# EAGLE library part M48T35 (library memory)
5V, 256 Kbit (32 Kb x8) TIMEKEEPER® SRAM Source: http://www.st.com/stonline/books/pdf/docs/2611.pdf#search=%22M48T35%22
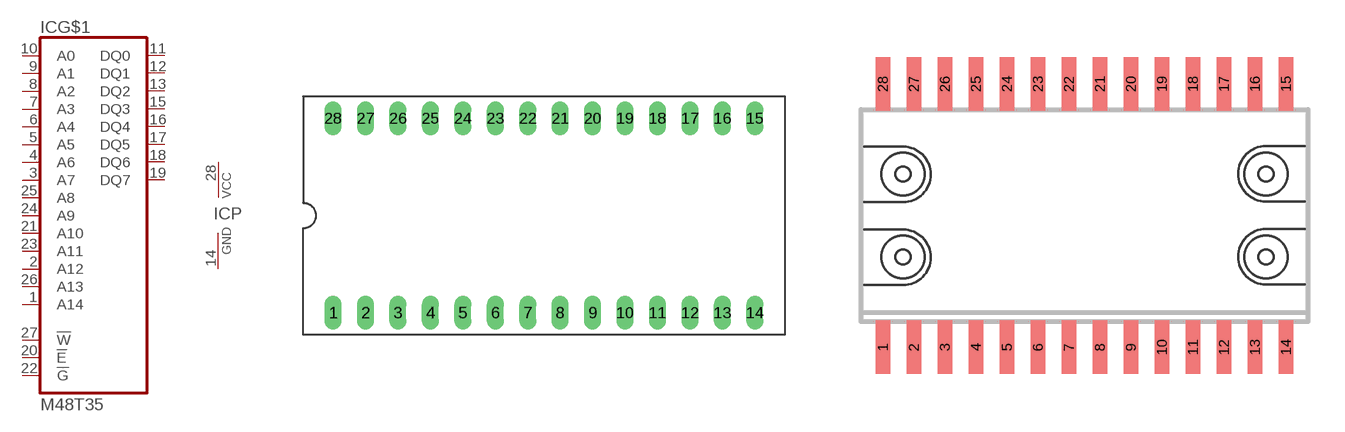
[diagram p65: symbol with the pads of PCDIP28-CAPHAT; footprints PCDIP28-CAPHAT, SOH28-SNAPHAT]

Designator prefix IC; gates G$1=M48T35 P=PWRN

## M48T35PC  [PCDIP28-CAPHAT]
1  G$1:A14  in
2  G$1:A12  in
3  G$1:A7  in
4  G$1:A6  in
5  G$1:A5  in
6  G$1:A4  in
7  G$1:A3  in
8  G$1:A2  in
9  G$1:A1  in
10  G$1:A0  in
11  G$1:DQ0
12  G$1:DQ1
13  G$1:DQ2
14  P:GND  pwr
15  G$1:DQ3
16  G$1:DQ4
17  G$1:DQ5
18  G$1:DQ6
19  G$1:DQ7
20  G$1:!E  in
21  G$1:A10  in
22  G$1:!G  in
23  G$1:A11  in
24  G$1:A9  in
25  G$1:A8  in
26  G$1:A13  in
27  G$1:!W  in
28  P:VCC  pwr

## M48T35MH  [SOH28-SNAPHAT]
Pads as for PCDIP28-CAPHAT

## Footprint PCDIP28-CAPHAT (pad centres in mm)
28-pin PCDIP, CAPHAT(TM) Package PCDIP28 (PC) Source: http://www.st.com/stonline/books/pdf/docs/2611.pdf#search=%22M48T35%22
drill 0.813 long: 1 -16.51,-7.62; 2 -13.97,-7.62; 3 -11.43,-7.62; 4 -8.89,-7.62; 5 -6.35,-7.62; 6 -3.81,-7.62; 7 -1.27,-7.62; 8 1.27,-7.62; 9 3.81,-7.62; 10 6.35,-7.62; 11 8.89,-7.62; 12 11.43,-7.62; 13 13.97,-7.62; 14 16.51,-7.62; 15 16.51,7.62; 16 13.97,7.62; 17 11.43,7.62; 18 8.89,7.62; 19 6.35,7.62; 20 3.81,7.62; 21 1.27,7.62; 22 -1.27,7.62; 23 -3.81,7.62; 24 -6.35,7.62; 25 -8.89,7.62; 26 -11.43,7.62; 27 -13.97,7.62; 28 -16.51,7.62

## Footprint SOH28-SNAPHAT (pad centres in mm)
28-pin SOH28 (MH) Source: http://www.st.com/stonline/books/pdf/docs/2611.pdf#search=%22M48T35%22
smd 0.6 x 2.2: 1 -8.255,-5.4; 2 -6.985,-5.4; 3 -5.715,-5.4; 4 -4.445,-5.4; 5 -3.175,-5.4; 6 -1.905,-5.4; 7 -0.635,-5.4; 8 0.635,-5.4; 9 1.905,-5.4; 10 3.175,-5.4; 11 4.445,-5.4; 12 5.715,-5.4; 13 6.985,-5.4; 14 8.255,-5.4; 15 8.255,5.4; 16 6.985,5.4; 17 5.715,5.4; 18 4.445,5.4; 19 3.175,5.4; 20 1.905,5.4; 21 0.635,5.4; 22 -0.635,5.4; 23 -1.905,5.4; 24 -3.175,5.4; 25 -4.445,5.4; 26 -5.715,5.4; 27 -6.985,5.4; 28 -8.255,5.4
